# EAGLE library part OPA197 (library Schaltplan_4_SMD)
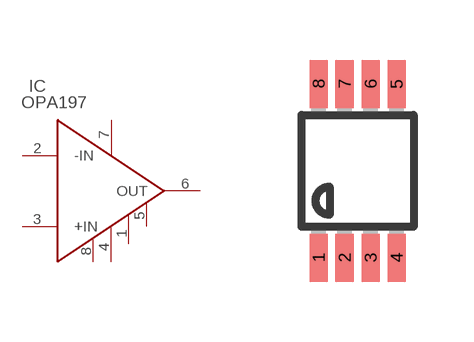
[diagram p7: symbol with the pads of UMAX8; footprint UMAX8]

Designator prefix IC

## OPA197  [UMAX8]
1  NC  nc
2  -IN  in
3  +IN  in
4  -V  pwr
5  NC  nc
6  OUT  out
7  +V  pwr
8  NC  nc

## Footprint UMAX8 (pad centres in mm)
micro MAX Package
smd 0.45 x 1.2: 1 -0.975,-2.175; 2 -0.325,-2.175; 3 0.325,-2.175; 4 0.975,-2.175; 5 0.975,2.175; 6 0.325,2.175; 7 -0.325,2.175; 8 -0.975,2.175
